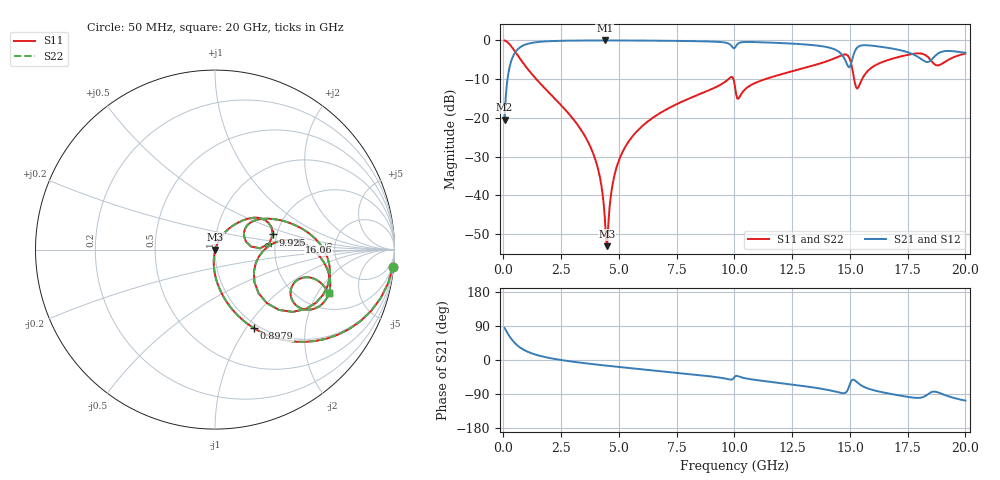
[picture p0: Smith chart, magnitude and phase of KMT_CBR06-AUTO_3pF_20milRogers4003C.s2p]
! Data measured by Modelithics Inc. support@modelithics.com 813-866-6335
! KEMET CBR06-AUTO 3pF, Pad Width= 0.851mm, Pad Length= 0.64mm, Pad Gap= 0.62mm, 20mil Rogers 4003C substrate Data, January 2022
# hz S ma R 50
! 2 Port Network Data from SP1.SP block
! freq  magS11  angS11  magS21  angS21  magS12  angS12  magS22  angS22
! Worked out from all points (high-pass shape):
!   401 points, 50 MHz to 20 GHz, reference 50 ohm
!   highest |S21| = -0.02 dB at 4.389 GHz (marker M1); lowest = -20.5 dB at 50 MHz (marker M2)
!   |S21| within 3 dB of the highest: 518.8 MHz to 14.54 GHz (14.02 GHz wide, 186 % of centre); 15.2 GHz to 17.48 GHz (2.279 GHz wide, 13.9 % of centre)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
!   lowest |S11| = -53.1 dB at 4.489 GHz (marker M3), VSWR 1.00, Z = 50.2 + j0.0315 ohm
!   |S11| at or under -10 dB: 1.422 GHz to 9.739 GHz (8.317 GHz wide, 149 % of centre); 9.955 GHz to 11.33 GHz (1.378 GHz wide, 13 % of centre); 15.18 GHz to 15.53 GHz (344.7 MHz wide, 2.24 % of centre)
!   |S22| runs from -53.1 to 0.0 dB; largest |S21 - S12| = 0
!   S11 on the Smith chart (normalised r, x): 50 MHz: 1, -20; 897.9 MHz: 0.95, -1.09; 9.925 GHz: 1.91, +0.36; 16.06 GHz: 2.73, +0.30; 20 GHz: 2.79, -2.51
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5e7  0.9955 -5.6  0.0949 84.4  0.0949 84.4  0.9955 -5.6
3.4925e8  0.8304 -35.0  0.5561 55.0  0.5561 55.0  0.8304 -35.0
8.97875e8  0.4895 -63.6  0.8709 26.3  0.8709 26.3  0.4895 -63.6
3.391625e9  0.0679 -96.0  0.9958 -7.5  0.9958 -7.5  0.0679 -96.0
4.089875e9  0.02221 -97.5  0.9977 -12.5  0.9977 -12.5  0.02221 -97.5
4.389125e9  0.005127 -81.3  0.9978 -14.5  0.9978 -14.5  0.005127 -81.3
4.488875e9  0.002217 8.1  0.9978 -15.1  0.9978 -15.1  0.002217 8.1
4.788125e9  0.01726 65.9  0.9976 -17.0  0.9976 -17.0  0.01726 65.9
5.13725e9  0.03536 67.2  0.997 -19.2  0.997 -19.2  0.03536 67.2
6.73325e9  0.1131 59.7  0.9907 -29.0  0.9907 -29.0  0.1131 59.7
9.92525e9  0.3334 14.7  0.813 -50.6  0.813 -50.6  0.3334 14.7
1.0025e10  0.2521 1.6  0.8058 -43.6  0.8058 -43.6  0.2521 1.6
1.02245e10  0.1867 30.0  0.9328 -44.3  0.9328 -44.3  0.1867 30.0
1.336662e10  0.4701 16.6  0.8706 -72.0  0.8706 -72.0  0.4701 16.6
1.471325e10  0.653 -11.3  0.6178 -87.6  0.6178 -87.6  0.653 -11.3
1.50125e10  0.5553 -38.7  0.4644 -61.7  0.4644 -61.7  0.5553 -38.7
1.531175e10  0.2394 -18.8  0.8044 -59.0  0.8044 -59.0  0.2394 -18.8
1.605988e10  0.4696 5.3  0.8473 -80.3  0.8473 -80.3  0.4696 5.3
1.670825e10  0.5649 -1.8  0.7954 -88.8  0.7954 -88.8  0.5649 -1.8
1.830425e10  0.6361 -31.5  0.5281 -93.5  0.5281 -93.5  0.6361 -31.5
1.875312e10  0.4768 -27.3  0.656 -84.3  0.656 -84.3  0.4768 -27.3
2e10  0.6778 -21.0  0.6902 -107.1  0.6902 -107.1  0.6778 -21.0
